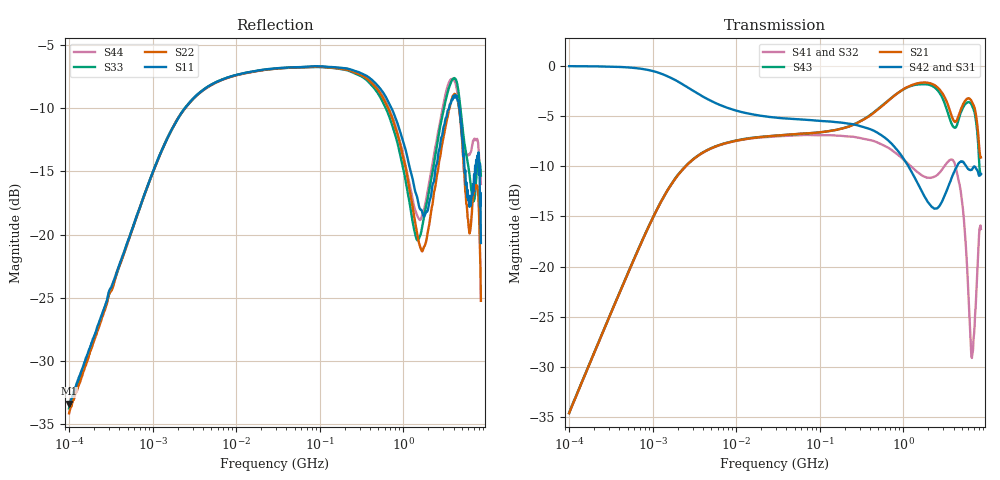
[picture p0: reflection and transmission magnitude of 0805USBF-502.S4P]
# Hz S dB R 50
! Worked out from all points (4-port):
!   801 points, 100 kHz to 8.5 GHz, reference 50 ohm
!   strongest paths, dB at 100 kHz, 1.721 MHz, 29.51 MHz, 502.3 MHz, 8.5 GHz:
!     S42: 0.0, -1.3, -5.2, -6.7, -10.8
!     S31: -0.1, -1.3, -5.2, -6.8, -12.5
!     S21: -34.6, -11.7, -7.0, -4.3, -9.1
!     S43: -34.6, -11.6, -7.0, -4.3, -10.8
!     S41: -34.6, -11.7, -7.0, -7.7, -16.3
!     S32: -34.7, -11.7, -7.1, -7.8, -18.6
!   lowest |S11| = -33.4 dB at 100 kHz (marker M1), VSWR 1.04, Z = 50.4 + j2.12 ohm
!   |S11| at or under -10 dB: start of sweep to 2.437 MHz; 724.5 MHz to 3.528 GHz (2.804 GHz wide, 132 % of centre); 4.689 GHz to end of sweep
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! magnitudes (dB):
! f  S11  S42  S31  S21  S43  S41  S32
! 100 kHz  -33.4  0.0  -0.1  -34.6  -34.6  -34.6  -34.7
! 7.992 MHz  -7.6  -4.2  -4.3  -7.6  -7.6  -7.7  -7.7
! 379.2 MHz  -7.5  -6.2  -6.3  -5.1  -5.1  -7.4  -7.5
! 1.501 GHz  -17.4  -11.8  -11.8  -1.7  -1.9  -10.6  -10.8
! 4.21 GHz  -9.0  -10.3  -9.9  -5.6  -6.2  -10.0  -10.3
! 6.635 GHz  -16.8  -10.4  -10.4  -3.6  -3.9  -29.1  -23.7
! 8.5 GHz  -20.7  -10.8  -12.5  -9.1  -10.8  -16.3  -18.6
